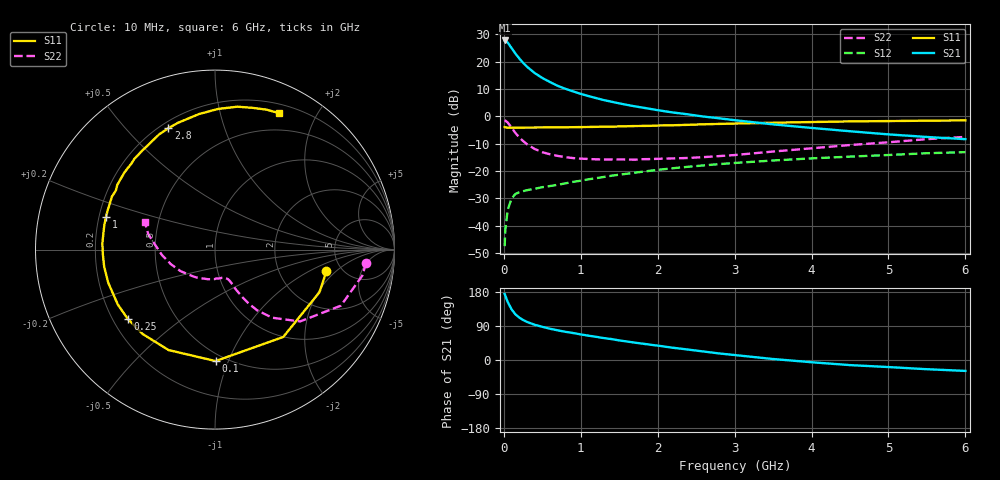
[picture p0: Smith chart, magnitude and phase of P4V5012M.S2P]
! SIEMENS Small Signal Semiconductors
! BFP182
! Si NPN RF Bipolar Junction Transistor in SOT143
! VCE = 0.5 V  IC = 12 mA
! Common Emitter S-Parameters:  March  1996
# GHz  S  MA  R  50
!  f  S11  S21  S12  S22
! GHz  MAG  ANG  MAG  ANG  MAG  ANG  MAG  ANG
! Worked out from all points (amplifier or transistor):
!   36 points, 10 MHz to 6 GHz, reference 50 ohm
!   highest |S21| = 27.7 dB at 10 MHz (marker M1)
!   |S21| within 3 dB of that: start of sweep to 106.1 MHz
!   unconditionally stable (mu >= 1): 416.7 MHz to end of sweep
!   at 250 MHz: K = 0.66, MSG = 23.5 dB, |S12| = -27.4 dB
!   at 1.4 GHz: K = 1.88, MAG = 8.1 dB, |S12| = -21.8 dB
!   at 6 GHz: K = 1.61, MAG = -2.2 dB, |S12| = -13.1 dB
!   S11 on the Smith chart (normalised r, x): 10 MHz: 3.78, -1.53; 100 MHz: 0.45, -0.90; 250 MHz: 0.26, -0.33; 1 GHz: 0.23, +0.14; 2.8 GHz: 0.23, +0.66; 6 GHz: 0.30, +1.54
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0.01  0.6323 -11.1  24.38 174.5  0.0042 81.7  0.8458 -5.0
0.02  0.6287 -22.2  24.35 169.1  0.0085 78.5  0.833 -10.1
0.05  0.6177 -52.0  22.34 153.2  0.0194 66.3  0.7679 -24.0
0.1  0.621 -89.7  17.76 133.9  0.0311 50.6  0.6202 -40.2
0.15  0.6166 -114.8  14.07 120.6  0.0379 41.7  0.4963 -49.9
0.2  0.6196 -130.7  11.45 112.0  0.0406 37.3  0.4111 -55.3
0.25  0.6207 -141.7  9.494 105.6  0.0426 34.4  0.3524 -58.1
0.3  0.6219 -150.6  8.078 100.6  0.0444 33.6  0.3088 -59.9
0.4  0.6227 -162.6  6.2 93.0  0.0471 33.1  0.2522 -62.3
0.5  0.6248 -171.2  5.014 87.5  0.0504 33.4  0.2202 -63.4
0.6  0.6254 -177.7  4.234 82.5  0.0529 34.8  0.2017 -64.1
0.7  0.6284 176.9  3.603 78.3  0.0557 36.3  0.1883 -65.2
0.8  0.6284 172.0  3.183 74.4  0.0592 37.3  0.1786 -66.6
1  0.6344 163.2  2.568 67.5  0.0663 39.0  0.1677 -70.1
1.1  0.6369 159.6  2.342 64.2  0.0703 39.5  0.1654 -72.3
1.5  0.6529 146.5  1.722 51.6  0.0853 40.3  0.1622 -81.3
2.2  0.6849 125.9  1.172 32.3  0.1121 37.5  0.1695 -103.4
2.8  0.7244 111.0  0.918 17.3  0.1333 32.8  0.1869 -123.9
3.5  0.7609 96.6  0.711 2.6  0.1552 26.8  0.2263 -147.9
4.5  0.8059 81.1  0.532 -13.5  0.1827 17.9  0.2976 -174.3
5.5  0.8306 69.9  0.418 -24.3  0.2108 9.3  0.3815 167.0
6  0.8407 64.7  0.381 -28.8  0.2204 4.1  0.4195 158.7
